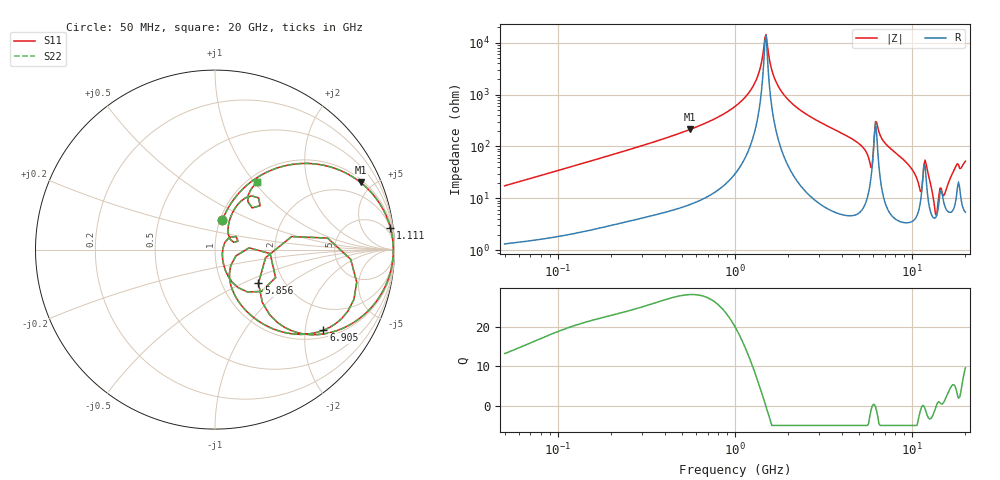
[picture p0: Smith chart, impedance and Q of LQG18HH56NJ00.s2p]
!Murata Part Number: LQG18HH56NJ00
!These Parameters are Measured in Series Mode Connection
!  o--[Z]--o
!Port1  Port2
!  o-------o
!Freq. Start=50[MHz] Stop=20[GHz], 401[Steps]
# Hz S RI R 50
!Freq.(Hz) S11(Real) S11(Imag) S21(Real) S21(Imag) S12(Real) S12(Imag) S22(Real) S22(Imag)
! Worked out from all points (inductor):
!   401 points, 50 MHz to 20 GHz, reference 50 ohm
!   read as one part in series: L = 54.8 nH near 51.52 MHz
!   highest Q = 28.1 at 557.6 MHz (marker M1), where L = 60.8 nH
!   self-resonance near 1.476 GHz
!   S11 on the Smith chart (normalised r, x): 50 MHz: 1.03, +0.35; 1.111 GHz: 2, +16; 5.856 GHz: 1.49, -0.61; 6.905 GHz: 1.21, -2.51; 20 GHz: 1.11, +1.03
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5e7  0.0412 0.1643  0.9588 -0.1643  0.9588 -0.1643  0.0412 0.1643
1.364002e8  0.1904 0.3694  0.8096 -0.3694  0.8096 -0.3694  0.1904 0.3694
3.721004e8  0.6291 0.4644  0.3709 -0.4644  0.3709 -0.4644  0.6291 0.4644
5.575697e8  0.8111 0.374  0.1889 -0.374  0.1889 -0.374  0.8111 0.374
1e9  0.9645 0.1616  0.0355 -0.1616  0.0355 -0.1616  0.9645 0.1616
1.110545e9  0.9776 0.1198  0.0224 -0.1198  0.0224 -0.1198  0.9776 0.1198
1.329223e9  0.9909 0.0471  0.00912 -0.0471  0.00912 -0.0471  0.9909 0.0471
1.498439e9  0.9934 -0.00194  0.00658 0.00194  0.00658 0.00194  0.9934 -0.00194
1.639343e9  0.992 -0.039  0.00799 0.039  0.00799 0.039  0.992 -0.039
1.793498e9  0.9876 -0.0764  0.0124 0.0764  0.0124 0.0764  0.9876 -0.0764
2.728004e9  0.9212 -0.2555  0.0788 0.2555  0.0788 0.2555  0.9212 -0.2555
5.117541e9  0.5311 -0.4737  0.4689 0.4737  0.4689 0.4737  0.5311 -0.4737
5.856089e9  0.2423 -0.1872  0.7577 0.1872  0.7577 0.1872  0.2423 -0.1872
6.311513e9  0.7897 -0.1821  0.2103 0.1821  0.2103 0.1821  0.7897 -0.1821
6.905011e9  0.6041 -0.4495  0.3959 0.4495  0.3959 0.4495  0.6041 -0.4495
7.442007e9  0.4781 -0.4723  0.5219 0.4723  0.5219 0.4723  0.4781 -0.4723
9.745021e9  0.1619 -0.3284  0.8381 0.3284  0.8381 0.3284  0.1619 -0.3284
1.115139e10  0.0879 -0.0879  0.9121 0.0879  0.9121 0.0879  0.0879 -0.0879
1.201863e10  0.2577 -0.2335  0.7423 0.2335  0.7423 0.2335  0.2577 -0.2335
1.354865e10  0.0409 -0.026  0.9591 0.026  0.9591 0.026  0.0409 -0.026
1.747767e10  0.1715 0.2892  0.8285 -0.2892  0.8285 -0.2892  0.1715 0.2892
2e10  0.2352 0.375  0.7648 -0.375  0.7648 -0.375  0.2352 0.375
